VAR_GLOBAL
	// 视觉变量
	// 坐标点（标定以及配方粗出用）
	aSrcPoint					:	ARRAY[0..8] OF TcVnPoint2_REAL :=[[967.9852,861.1947],[639.944,861.18853],[311.5,860.801],[967.622,532.9594],[639.644,532.828],[311.864,532.829],[967.319,205.2013],[639.450,204.844],[311.7406,205.044]];	// 9点像素坐标
	aDestPoint					:	ARRAY[0..8] OF TcVnPoint2_REAL :=[[-41.25,-205.59],[-41.029,-163.918],[-40.057,-122.651],[0,-205.59],[0.5,-163.918],[1.513,-122.651],[41.017,-205.59],[41.989,-165.25],[42.846,-122.651]];	// 9点机器人坐标
	srcpoint					:	ARRAY[0..8, 0..1] OF REAL;
	destpoint					:	ARRAY[0..8, 0..1] OF REAL;
	// 坐标变换矩阵
	aTransformationMatrix		:	TcVnMatrix3x3_LREAL;
	// 错误标志位以及错误信息
	bVisionErr					:	BOOL;// 视觉系统报警
	VisionErrMessage			:	WSTRING(255);// 报警信息
	bVisionWarning				:	BOOL;// warning（依旧可以正常运行）
	// 有效提取图像
	bGetImage					:	BOOL;// 是否成功提取到图片
	// 视觉系统就绪标志位
	VisionReady					:	BOOL;// 视觉系统就绪后置位
	// 启用视觉系统
	VisionStartPush				:	BOOL;// 置位后开启抓取模式
	// 物料结构体
	dmaterial					:	DUT_material;
	// 视觉暂停
	VisionHalt					:	BOOL;
	// 队列系统
	gArrayStmaterial				:	ARRAY[1..INUM] OF DUT_material;
	gStmaterialNULL			:	DUT_material;
	gbPushPopBusy				:	BOOL;		
	gfbPushPopStack				:	FB_PushPopStack;	
//	gfbPushStack				:	FB_PushStack;
//	gfbPopStack					:	FB_PopStack;
	// 皮带偏移
	lrBeltOffset				:	LREAL  := 466.5;
END_VAR

VAR_GLOBAL CONSTANT
	INUM	:INT:=30;
END_VAR
